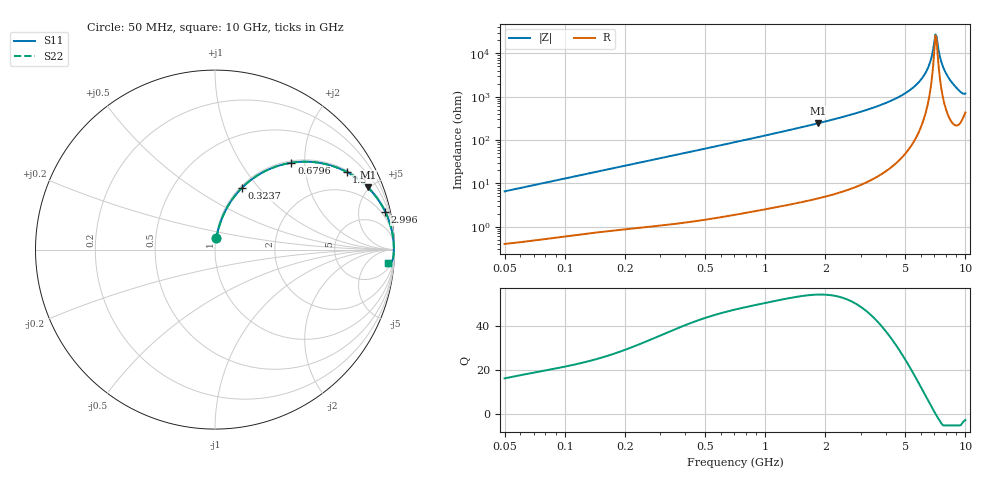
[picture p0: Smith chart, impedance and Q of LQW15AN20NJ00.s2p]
!Murata Part Number: LQW15AN20NJ00
!These Parameters are Measured in Series Mode Connection
!  o--[Z]--o
!Port1  Port2
!  o-------o
!Freq. Start=50[MHz] Stop=10[GHz], 401[Steps]
# Hz S RI R 50
!Freq.(Hz)	S 11(Real)	S 11(Imag)	S 21(Real)	S 21(Imag)	S 12(Real)	S 12(Imag)	S 22(Real)	S 22(Imag)
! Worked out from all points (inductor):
!   401 points, 50 MHz to 10 GHz, reference 50 ohm
!   read as one part in series: L = 20.7 nH near 51.34 MHz
!   highest Q = 54.3 at 1.835 GHz (marker M1), where L = 21.1 nH
!   self-resonance near 7.087 GHz
!   S11 on the Smith chart (normalised r, x): 50 MHz: 1.01, +0.13; 323.7 MHz: 1.02, +0.82; 679.6 MHz: 1.04, +1.72; 1.3 GHz: 1.06, +3.34; 2.996 GHz: 1.18, +8.95; 10 GHz: 10, -22
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5e7  0.00819 0.0646  0.9918 -0.0646  0.9918 -0.0646  0.00819 0.0646
1.214486e8  0.0299 0.1502  0.9701 -0.1502  0.9701 -0.1502  0.0299 0.1502
2.949953e8  0.1292 0.3216  0.8708 -0.3216  0.8708 -0.3216  0.1292 0.3216
3.236556e8  0.1501 0.3439  0.8499 -0.3439  0.8499 -0.3439  0.1501 0.3439
6.795592e8  0.4259 0.484  0.5741 -0.484  0.5741 -0.484  0.4259 0.484
7.071068e8  0.4452 0.4866  0.5548 -0.4866  0.5548 -0.4866  0.4452 0.4866
1.300479e9  0.7326 0.4332  0.2674 -0.4332  0.2674 -0.4332  0.7326 0.4332
1.717543e9  0.8317 0.3651  0.1683 -0.3651  0.1683 -0.3651  0.8317 0.3651
1.835145e9  0.851 0.347  0.149 -0.347  0.149 -0.347  0.851 0.347
2.99582e9  0.9486 0.2108  0.0514 -0.2108  0.0514 -0.2108  0.9486 0.2108
4.171863e9  0.9802 0.1258  0.0198 -0.1258  0.0198 -0.1258  0.9802 0.1258
5.225452e9  0.9915 0.072  0.00853 -0.072  0.00853 -0.072  0.9915 0.072
6.045081e9  0.9953 0.0382  0.00472 -0.0382  0.00472 -0.0382  0.9953 0.0382
6.54512e9  0.9963 0.0197  0.0037 -0.0197  0.0037 -0.0197  0.9963 0.0197
6.720828e9  0.9965 0.0136  0.00353 -0.0136  0.00353 -0.0136  0.9965 0.0136
6.993273e9  0.9965 0.00424  0.00345 -0.00424  0.00345 -0.00424  0.9965 0.00424
7.086521e9  0.9965 0.00111  0.00347 -0.00111  0.00347 -0.00111  0.9965 0.00111
7.276762e9  0.9964 -0.00518  0.00359 0.00518  0.00359 0.00518  0.9964 -0.00518
7.672705e9  0.9958 -0.018  0.00419 0.018  0.00419 0.018  0.9958 -0.018
8.090191e9  0.9946 -0.0312  0.00538 0.0312  0.00538 0.0312  0.9946 -0.0312
9.114482e9  0.9867 -0.0634  0.0133 0.0634  0.0133 0.0634  0.9867 -0.0634
1e10  0.9646 -0.0735  0.0354 0.0735  0.0354 0.0735  0.9646 -0.0735
